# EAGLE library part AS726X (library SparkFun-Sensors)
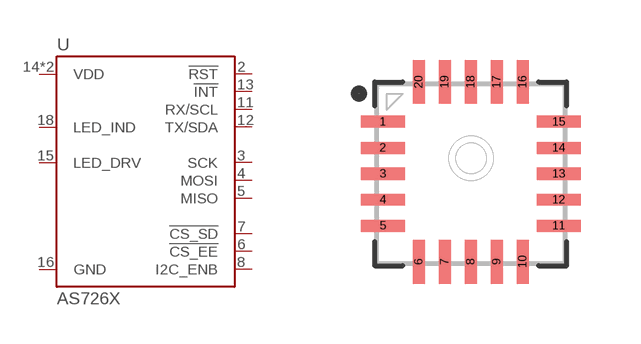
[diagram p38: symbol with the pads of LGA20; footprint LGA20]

Designator prefix U

## AS726XIR (PROD_ID: IC-13731; VALUE: IR)  [LGA20]
2  !RST
3  SCK
4  MOSI
5  MISO
6  !CS_EE
7  !CS_SD
8  I2C_ENB
11  RX/SCL
12  TX/SDA
13  !INT
14  VDD
15  LED_DRV
16  GND
17  VDD
18  LED_IND

## AS726XVISIBLE (PROD_ID: IC_13724; VALUE: VISIBLE)  [LGA20]
Pads as for LGA20

## Footprint LGA20 (pad centres in mm)
smd 1.1 x 0.3: 1 -2.2,1.3; 2 -2.2,0.65; 3 -2.2,0; 4 -2.2,-0.65; 5 -2.2,-1.3; 11 2.2,-1.3; 12 2.2,-0.65; 13 2.2,0; 14 2.2,0.65; 15 2.2,1.3
smd 0.3 x 1.1: 6 -1.3,-2.2; 7 -0.65,-2.2; 8 0,-2.2; 9 0.65,-2.2; 10 1.3,-2.2; 16 1.3,2.3; 17 0.65,2.3; 18 0,2.3; 19 -0.65,2.3; 20 -1.3,2.3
